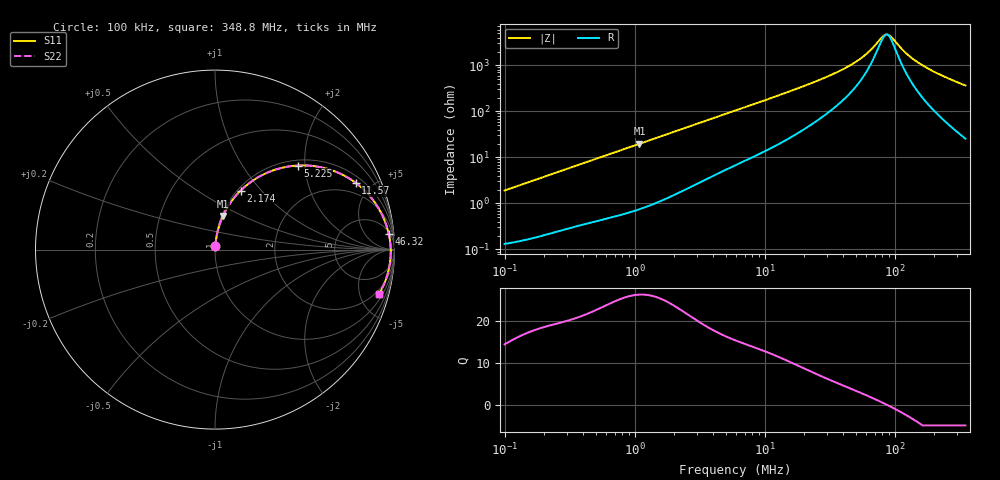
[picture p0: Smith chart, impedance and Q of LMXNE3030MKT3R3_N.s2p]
! LMXNE3030MKT3R3_N  S-PARAMETER MODEL  ( General Type )
! Model Generated by TAIYO YUDEN Corporation (http://www.ty-top.com)
! Version 1.0
! TAIYO YUDEN Control No. 191023NI43SB-FBB
! Copyright(c) 2019 TAIYO YUDEN CO.,LTD. All Rights Reserved.
! Product Description (link to TY-COMPAS)
! https://ds.yuden.co.jp/TYCOMPAS/or/detail?pn=LMXNE3030MKT3R3MN&u=M
! Products Name : Inductors
! Characteristics :
!  Inductance : 3.3 uH , SRF(min) : 61 MHz , DC Resistance(max) : 0.12 Ohm
!  Rated Current : Saturation :1200 mA , Temp Rise : 1210 mA
!  Case Size : 3.0 x 3.0 / 0.118 x 0.118 [mm/inch] , Thickness : 1.2 / 0.047 [mm/inch]
!  (Conditions: Temperature = 25 degC , DC Bias Current/Voltage = 0A / 0V)
! External Node Assignments :
!  1  o---GGG---o  2
! GND o---------o GND
! Frequency Range : 0.1MHz  -  348.750116MHz  [ 402 STEP ]
# MHz S RI R 50
! Freq[MHz].  S11 Real  S11 Imag  S21 Real  S21 Imag  S12 Real  S12 Imag  S22 Real  S22 Imag
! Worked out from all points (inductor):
!   401 points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, 100 kHz to 348.8 MHz, reference 50 ohm
!   read as one part in series: L = 3.02 uH near 104.2 kHz
!   highest Q = 26.4 at 1.087 MHz (marker M1), where L = 2.88 uH
!   self-resonance near 86.36 MHz
!   S11 on the Smith chart (normalised r, x): 100 kHz: 1.00, +0.04; 2.174 MHz: 1.03, +0.78; 5.225 MHz: 1.11, +1.84; 11.57 MHz: 1.33, +4.01; 46.32 MHz: 6, +20; 348.8 MHz: 1.51, -7.28
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0.1  0.00167 0.019  0.9983 -0.019  0.9983 -0.019  0.00167 0.019
0.392077  0.00858 0.0716  0.9914 -0.0716  0.9914 -0.0716  0.00858 0.0716
1.08689  0.044 0.187  0.956 -0.187  0.956 -0.187  0.044 0.187
1.537242  0.08 0.2525  0.92 -0.2525  0.92 -0.2525  0.08 0.2525
2.174198  0.1429 0.329  0.8571 -0.329  0.8571 -0.329  0.1429 0.329
3.269075  0.2639 0.4158  0.7361 -0.4158  0.7361 -0.4158  0.2639 0.4158
5.225399  0.4606 0.4684  0.5394 -0.4684  0.5394 -0.4684  0.4606 0.4684
5.905507  0.5166 0.4684  0.4834 -0.4684  0.4834 -0.4684  0.5166 0.4684
8.018654  0.6512 0.442  0.3488 -0.442  0.3488 -0.442  0.6512 0.442
11.57483  0.7835 0.3723  0.2165 -0.3723  0.2165 -0.3723  0.7835 0.3723
16.0404  0.865 0.2957  0.135 -0.2957  0.135 -0.2957  0.865 0.2957
23.15412  0.9213 0.2125  0.0787 -0.2125  0.0787 -0.2125  0.9213 0.2125
34.11126  0.9538 0.1378  0.0462 -0.1378  0.0462 -0.1378  0.9538 0.1378
46.31717  0.9679 0.0879  0.0321 -0.0879  0.0321 -0.0879  0.9679 0.0879
61.62119  0.9754 0.0464  0.0246 -0.0464  0.0246 -0.0464  0.9754 0.0464
81.98192  0.9789 0.0071  0.0211 -0.0071  0.0211 -0.0071  0.9789 0.0071
87.15392  0.9792 -0.00125  0.0208 0.00125  0.0208 0.00125  0.9792 -0.00125
90.78195  0.9793 -0.00684  0.0207 0.00684  0.0207 0.00684  0.9793 -0.00684
120.7779  0.9779 -0.0469  0.0221 0.0469  0.0221 0.0469  0.9779 -0.0469
154.2634  0.9734 -0.0841  0.0266 0.0841  0.0266 0.0841  0.9734 -0.0841
222.6774  0.9581 -0.1483  0.0419 0.1483  0.0419 0.1483  0.9581 -0.1483
348.7501  0.9154 -0.2455  0.0846 0.2455  0.0846 0.2455  0.9154 -0.2455
